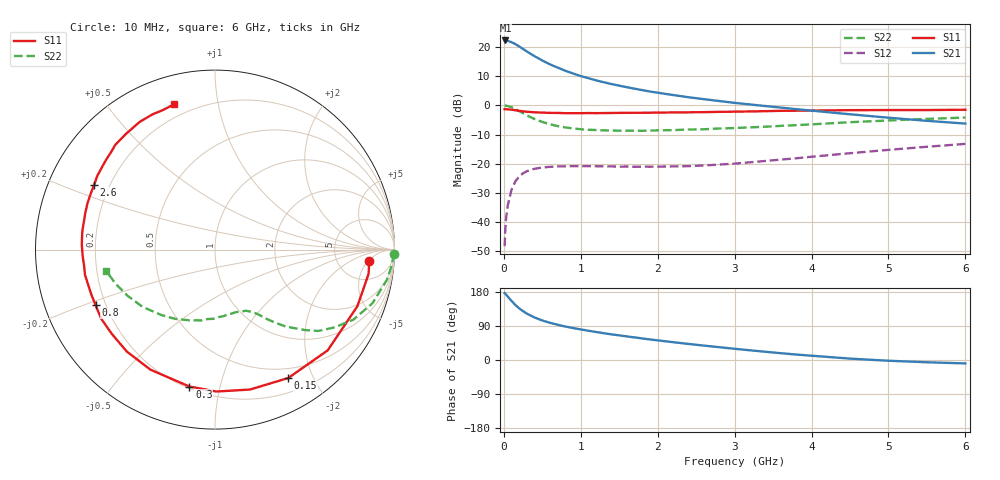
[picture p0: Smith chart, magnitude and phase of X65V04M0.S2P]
! SIEMENS Small Signal Semiconductors
! BFP193W
! Si NPN RF Bipolar Junction Transistor in SOT343
! VCE = 5 V  IC = 4 mA
! Common Emitter S-Parameters:  April 1994
# GHz  S  MA  R  50
!  f  S11  S21  S12  S22
! GHz  MAG  ANG  MAG  ANG  MAG  ANG  MAG  ANG
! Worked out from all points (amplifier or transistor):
!   40 points, 10 MHz to 6 GHz, reference 50 ohm
!   highest |S21| = 22.2 dB at 20 MHz (marker M1)
!   |S21| within 3 dB of that: start of sweep to 255.5 MHz
!   unconditionally stable (mu >= 1): 1.808 GHz to 4.382 GHz
!   at 200 MHz: K = 0.12, MSG = 22.2 dB, |S12| = -24.3 dB
!   at 1.5 GHz: K = 0.85, MSG = 13.8 dB, |S12| = -21.0 dB
!   at 6 GHz: K = 0.91, MSG = 3.5 dB, |S12| = -13.2 dB
!   S11 on the Smith chart (normalised r, x): 10 MHz: 11, -5; 150 MHz: 0.37, -1.66; 300 MHz: 0.21, -0.81; 800 MHz: 0.16, -0.22; 2.6 GHz: 0.14, +0.25; 6 GHz: 0.14, +0.75
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0.01  0.8616 -4.3  12.81 176.7  0.0039 89.5  0.9972 -1.3
0.02  0.8664 -8.9  12.86 175.0  0.0079 84.9  0.9901 -4.2
0.05  0.8537 -21.7  12.68 167.6  0.0192 78.8  0.9725 -10.0
0.1  0.8423 -41.8  12 155.9  0.036 68.1  0.927 -18.8
0.15  0.8237 -60.3  11.15 145.2  0.05 59.4  0.8637 -26.9
0.2  0.8036 -76.0  10.14 136.3  0.0607 51.8  0.7952 -33.0
0.25  0.7908 -89.4  9.209 128.9  0.0688 45.4  0.733 -38.2
0.3  0.776 -100.6  8.323 122.4  0.0747 40.5  0.6724 -41.8
0.4  0.7596 -118.3  6.911 112.2  0.0822 33.1  0.5825 -47.4
0.5  0.7509 -130.9  5.839 104.3  0.0864 28.2  0.5195 -51.0
0.6  0.7424 -140.8  5.019 98.1  0.0887 24.5  0.4738 -53.8
0.7  0.7417 -148.7  4.415 93.0  0.0901 22.2  0.4413 -55.7
0.8  0.7339 -155.0  3.894 88.3  0.0906 20.3  0.4188 -57.7
1.1  0.7379 -169.0  2.908 77.1  0.0913 17.6  0.3817 -63.1
1.3  0.7374 -176.4  2.477 70.7  0.0905 17.2  0.3731 -67.2
1.6  0.7441 174.7  2.04 62.1  0.0898 18.5  0.3676 -73.3
2.2  0.7556 160.3  1.5 47.0  0.0901 24.3  0.3767 -86.8
2.6  0.7638 151.9  1.274 38.0  0.0936 29.5  0.3894 -96.3
3.2  0.7863 140.6  1.035 25.6  0.106 36.5  0.4195 -110.3
4.5  0.8259 120.6  0.703 3.7  0.1517 42.0  0.5142 -141.6
5.5  0.8299 110.6  0.543 -6.0  0.1955 39.2  0.5859 -161.1
6  0.8406 105.9  0.487 -9.0  0.2191 37.0  0.6178 -168.9
